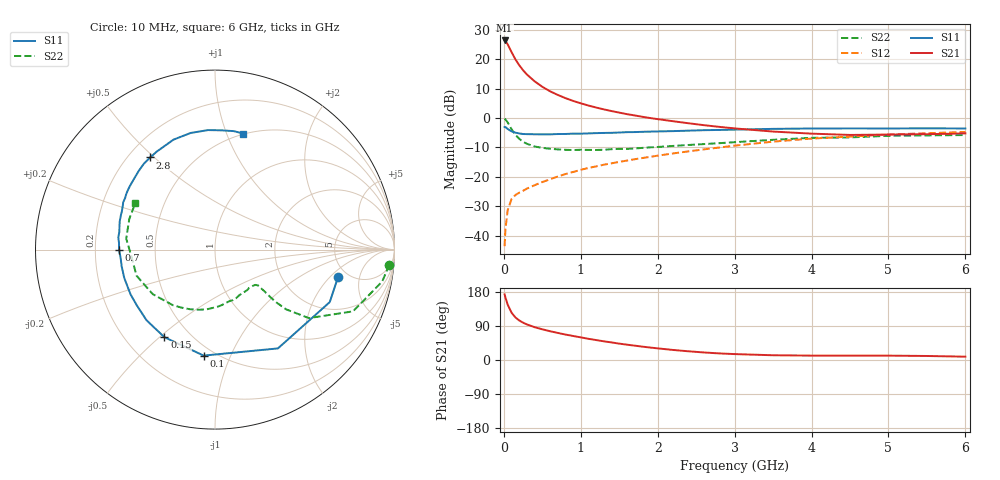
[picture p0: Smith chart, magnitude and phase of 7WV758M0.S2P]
! Infineon Technologies  Discrete & RF Semiconductors
! BFS17W
! Si NPN RF Bipolar Junction Transistor in SOT323
! VCE = 0.75 V  IC = 8 mA
! Common Emitter S-Parameters:  August  1999
# GHz  S  MA  R  50
!  f  S11  S21  S12  S22
! GHz  MAG  ANG  MAG  ANG  MAG  ANG  MAG  ANG
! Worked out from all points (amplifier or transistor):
!   36 points, 10 MHz to 6 GHz, reference 50 ohm
!   highest |S21| = 26.4 dB at 10 MHz (marker M1)
!   |S21| within 3 dB of that: start of sweep to 81.86 MHz
!   unconditionally stable (mu >= 1): 368.5 MHz to end of sweep
!   at 250 MHz: K = 0.81, MSG = 20.5 dB, |S12| = -24.8 dB
!   at 1.4 GHz: K = 1.35, MAG = 5.3 dB, |S12| = -15.4 dB
!   at 6 GHz: K = 1.13, MAG = -2.4 dB, |S12| = -4.7 dB
!   S11 on the Smith chart (normalised r, x): 10 MHz: 4.14, -2.50; 100 MHz: 0.44, -0.80; 150 MHz: 0.36, -0.52; 700 MHz: 0.30, -0.00; 2.8 GHz: 0.29, +0.49; 6 GHz: 0.49, +1.15
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0.01  0.7024 -12.6  20.93 173.1  0.0066 83.4  0.9746 -5.0
0.02  0.703 -24.6  20.49 165.3  0.0125 78.2  0.9485 -10.8
0.05  0.6527 -57.5  17.97 146.0  0.0272 64.7  0.8425 -24.1
0.1  0.594 -96.1  13.28 125.0  0.0417 51.6  0.6478 -36.1
0.15  0.5636 -120.0  10.02 112.4  0.049 46.1  0.5186 -40.0
0.2  0.5482 -134.1  7.936 104.4  0.0538 45.6  0.444 -40.8
0.25  0.535 -144.5  6.515 98.5  0.0578 45.4  0.3943 -40.5
0.3  0.5326 -152.0  5.515 93.9  0.063 46.9  0.3648 -40.2
0.4  0.5297 -162.7  4.216 86.6  0.0719 49.4  0.3276 -39.9
0.5  0.5283 -169.9  3.409 81.0  0.0814 52.0  0.3114 -39.8
0.6  0.5282 -175.4  2.858 76.0  0.0907 53.9  0.2997 -41.0
0.7  0.5345 -179.8  2.478 71.5  0.1012 55.2  0.2931 -43.2
0.9  0.5431 172.7  1.958 63.4  0.1208 56.9  0.2856 -48.6
1.1  0.5484 166.1  1.633 55.9  0.1415 57.3  0.2872 -55.3
1.3  0.5582 160.1  1.405 49.3  0.1608 57.4  0.289 -62.9
1.6  0.5756 152.6  1.166 40.5  0.1888 57.3  0.2985 -74.4
2.2  0.5995 138.6  0.883 26.5  0.2499 55.9  0.3356 -97.7
2.8  0.6277 125.1  0.708 17.4  0.315 52.5  0.3737 -120.3
3.5  0.6548 110.7  0.589 12.5  0.397 46.3  0.4266 -144.4
4.5  0.667 93.3  0.516 11.6  0.4833 34.4  0.4683 -175.9
5.5  0.6683 81.0  0.531 10.6  0.5518 23.8  0.507 160.4
6  0.6656 76.3  0.548 8.8  0.5803 18.8  0.5138 150.0
